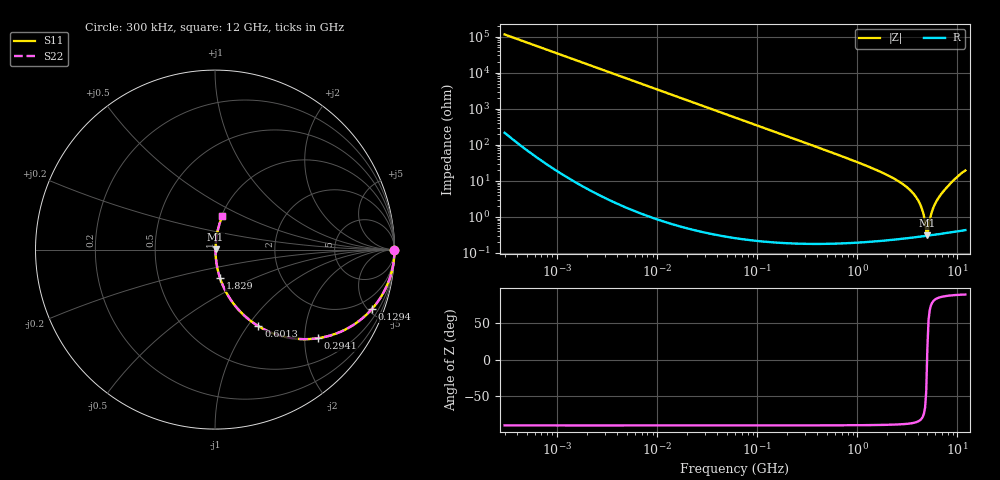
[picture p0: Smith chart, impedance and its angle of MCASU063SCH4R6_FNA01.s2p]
! MCASU063SCH4R6_FNA01  S-PARAMETER MODEL  ( General Type )
! Model Generated by TAIYO YUDEN Corporation (http://www.ty-top.com)
! Version 1.0
! TAIYO YUDEN Control No. 130801
! Copyright(c) 2013 TAIYO YUDEN CO.,LTD. All Rights Reserved.
! Product Description (link to TY-COMPAS)
! https://ds.yuden.co.jp/TYCOMPAS/or/detail?pn=MCASU063SCH4R6CFNA01&u=M
! Products Name : Multilayer Ceramic Capacitors
! Characteristics :
!  Capacitance : 4.6 pF , Rated Voltage : 50V , TCC : CH / C0H
!  Case Size : 0.6 x 0.3 / 0.024 x 0.012 [mm/inch] , Thickness : 0.3 / 0.012 [mm/inch]
!  (Conditions: Temperature = 25 degC , DC Bias Current/Voltage = 0A / 0V)
! External Node Assignments :
!  1  o---| |---o  2
! GND o---------o GND
! Frequency Range : 0.3MHz  -  12000MHz  [ 401 STEP ]
# MHz S RI R 50
! Freq[MHz].  S11 Real  S11 Imag  S21 Real  S21 Imag  S12 Real  S12 Imag  S22 Real  S22 Imag
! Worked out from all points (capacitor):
!   401 points, 300 kHz to 12 GHz, reference 50 ohm
!   read as one part in series: C = 4.63 pF near 316.3 kHz
!   lowest |Z| = 313 mohm at 5.006 GHz (marker M1)
!   series resonance near 4.977 GHz, so ESL is about 220 pH
!   S11 on the Smith chart (normalised r, x): 300 kHz: open; 129.4 MHz: 1.00, -5.31; 294.1 MHz: 1.00, -2.33; 601.3 MHz: 1.00, -1.13; 1.829 GHz: 1.00, -0.32; 12 GHz: 1.01, +0.39
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0.3  1 -0.000873  2.4e-06 0.000873  2.4e-06 0.000873  1 -0.000873
1.769972  1 -0.00515  2.85e-05 0.00515  2.85e-05 0.00515  1 -0.00515
10.44266  0.9991 -0.0304  0.000931 0.0304  0.000931 0.0304  0.9991 -0.0304
60  0.9703 -0.1695  0.0297 0.1695  0.0297 0.1695  0.9703 -0.1695
129.3602  0.8755 -0.3298  0.1245 0.3298  0.1245 0.3298  0.8755 -0.3298
294.0765  0.5753 -0.4935  0.4247 0.4935  0.4247 0.4935  0.5753 -0.4935
353.9943  0.4825 -0.4988  0.5175 0.4988  0.5175 0.4988  0.4825 -0.4988
601.3112  0.2414 -0.4263  0.7586 0.4263  0.7586 0.4263  0.2414 -0.4263
994.7115  0.1004 -0.2977  0.8996 0.2977  0.8996 0.2977  0.1004 -0.2977
1829.429  0.0277 -0.1576  0.9723 0.1576  0.9723 0.1576  0.0277 -0.1576
2088.533  0.0202 -0.1325  0.9798 0.1325  0.9798 0.1325  0.0202 -0.1325
2947.191  0.00816 -0.0749  0.9918 0.0749  0.9918 0.0749  0.00816 -0.0749
3740.715  0.00429 -0.0397  0.9957 0.0397  0.9957 0.0397  0.00429 -0.0397
4270.516  0.00329 -0.0211  0.9967 0.0211  0.9967 0.0211  0.00329 -0.0211
4502.883  0.00308 -0.0138  0.9969 0.0138  0.9969 0.0138  0.00308 -0.0138
4747.894  0.00299 -0.0065  0.997 0.0065  0.997 0.0065  0.00299 -0.0065
5006.236  0.00301 0.00082  0.997 -0.00082  0.997 -0.00082  0.00301 0.00082
5140.631  0.00305 0.00411  0.9969 -0.00411  0.9969 -0.00411  0.00305 0.00411
5715.274  0.00345 0.017  0.9965 -0.017  0.9965 -0.017  0.00345 0.017
6524.734  0.00453 0.0346  0.9955 -0.0346  0.9955 -0.0346  0.00453 0.0346
8966.534  0.0132 0.0964  0.9868 -0.0964  0.9868 -0.0964  0.0132 0.0964
12000  0.0402 0.1857  0.9598 -0.1857  0.9598 -0.1857  0.0402 0.1857
